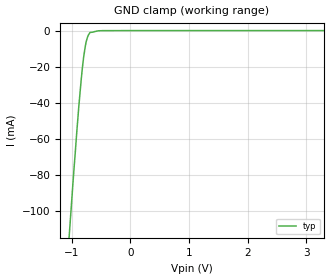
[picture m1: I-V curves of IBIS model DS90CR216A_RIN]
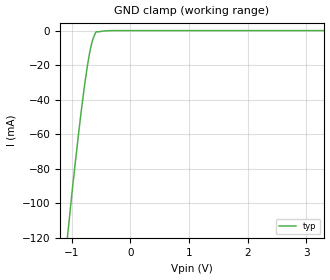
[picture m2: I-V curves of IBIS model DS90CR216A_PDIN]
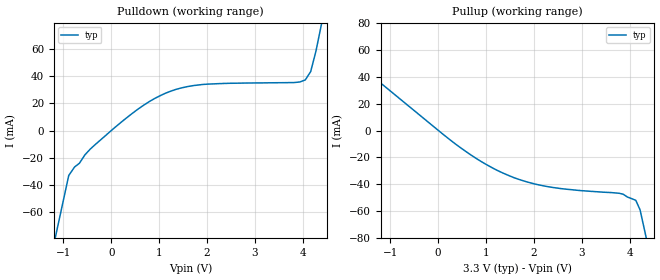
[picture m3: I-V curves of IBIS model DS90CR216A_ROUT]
|   National Semiconductor Corporation
|   Interface Products Group
|   IBIS Model of DS90CR216A
|   21-Bit LVDS Channel Link Receiver
|   48L TSSOP
[IBIS Ver]   2.1
[Comment char]  |_char
[File name]   90cr216a.ibs
[File Rev]   1.0
[Date]   10/07/04
[Source]   This is an empirical model.
[Notes]   File created by dglisic.
Rev. 1.0:
[Disclaimer]
(C) Copyright National Semiconductor Corporation 1994
   All rights reserved
   National Semiconductor Corporation hereby grants
the user of this IBIS model a non-exclusive, nontransferable
license to use this IBIS model under the following terms.
Before using this IBIS model, the user should read this
license.  If the user does not accept these terms,  the
IBIS model should be returned to National within 30 days.
   The user is granted this license only to use the
IBIS model and is not granted rights to sell, load, rent,
lease or license the IBIS model in whole or in part, or in
modified form to anyone other than user. User may modify
the IBIS model to suit its specific applications but rights
to derivative works and such modifications shall belong to
National.
   This IBIS model is provided on an "AS IS" basis and
National makes absolutely no warranty with respect to the
information contained herein.NATIONAL DISCLAIMS AND CUSTOMER
WAIVES ALL WARRANTIES, EXPRESS OR IMPLIED, INCLUDING
WARRANTIES OF MERCHANTABILITY OR FITNESS FOR A PARTICULAR
PURPOSE. The entire risk as to quality and performance is
with the Customer. ACCORDINGLY, IN NO EVENT SHALL THE
COMPANY BE LIABLE FOR ANY DAMAGES, WHETHER IN CONTRACT OR
TORT,INCLUDING ANY LOST PROFITS OR OTHER INCIDENTAL,
CONSEQUENTIAL, EXEMPLARY, OR PUNITIVE DAMAGES ARISING OUT
OF THE USE OR APPLICATION OF THE IBIS model provided in
this package.Further, National reserves the right to make
changes without notice to any product herein to improve
reliability, function, or design. National does not convey
any license under patent rights or any other intellectual
property rights, including those of third parties.
   National is not obligated to provide maintenance or support
for the licensed IBIS model.
Contact National at ATTN:INTERFACE APPLICATIONS/IBIS MODELS.
2900 Semiconductor Drive, M/S A2595, Santa Clara, CA 95052-8090
[Copyright]   Copyright 1994, National Semiconductor, All Rights Reserved
[Component]   DS90CR216AMTD
[Manufacturer]  National Semiconductor Corp
[Package]
|   typ   min   max
R_pkg   50.0m   50.0m   50.0m
L_pkg   1.49n   0.95n   2.07n
C_pkg   0.306p   0.146p   0.429p
[Pin]   signal_name   model_name   R_pin   L_pin   C_pin
1   RxOUT17   DS90CR216A_ROUT   50.0m   2.07n   0.429p
2   RxOUT18   DS90CR216A_ROUT   50.0m   1.49n   0.306p
3   GND   GND   50.0m   1.49n   0.146p
4   RxOUT19   DS90CR216A_ROUT   50.0m   0.95n   0.152p
5   RxOUT20   DS90CR216A_ROUT   50.0m   0.95n   0.152p
6   N/C   NC   50.0m   0.95n   0.146p
7   LVDSGND   GND   50.0m   1.49n   0.306p
8   RxIN0-   DS90CR216A_RIN   50.0m   2.07n   0.429p
9   RxIN0+   DS90CR216A_RIN   50.0m   2.07n   0.429p
10   RxIN1-   DS90CR216A_RIN   50.0m   1.49n   0.306p
11   RxIN1+   DS90CR216A_RIN   50.0m   0.95n   0.146p
12   LVDSVCC   POWER   50.0m   0.95n   0.152p
13   LVDSGND   GND   50.0m   0.95n   0.152p
14   RxIN2-   DS90CR216A_RIN   50.0m   0.95n   0.146p
15   RxIN2+   DS90CR216A_RIN   50.0m   1.49n   0.306p
16   RxCLKIN-   DS90CR216A_RIN   50.0m   2.07n   0.429p
17   RxCLKIN+   DS90CR216A_RIN   50.0m   2.07n   0.429p
18   LVDSGND   GND   50.0m   1.49n   0.306p
19   PLLGND   GND   50.0m   0.95n   0.146p
20   PLLVCC   POWER   50.0m   0.95n   0.152p
21   PLLGND   GND   50.0m   0.95n   0.152p
22   PWRDWN*   DS90CR216A_PDIN   50.0m   0.95n   0.146p
23   RxCLKOUT   DS90CR216A_ROUT   50.0m   1.49n   0.306p
24   RxOUT0   DS90CR216A_ROUT   50.0m   2.07n   0.429p
25   GND   GND   50.0m   2.07n   0.429p
26   RxOUT1   DS90CR216A_ROUT   50.0m   1.49n   0.306p
27   RxOUT2   DS90CR216A_ROUT   50.0m   0.95n   0.146p
28   VCC   POWER   50.0m   0.95n   0.152p
29   RxOUT3   DS90CR216A_ROUT   50.0m   0.95n   0.152p
30   RxOUT4   DS90CR216A_ROUT   50.0m   0.95n   0.146p
31   RxOUT5   DS90CR216A_ROUT   50.0m   1.49n   0.306p
32   GND   GND   50.0m   2.07n   0.429p
33   RxOUT6   DS90CR216A_ROUT   50.0m   2.07n   0.429p
34   RxOUT7   DS90CR216A_ROUT   50.0m   1.49n   0.306p
35   RxOUT8   DS90CR216A_ROUT   50.0m   0.95n   0.146p
36   VCC   POWER   50.0m   0.95n   0.152p
37   RxOUT9   DS90CR216A_ROUT   50.0m   0.95n   0.152p
38   GND   GND   50.0m   0.95n   0.146p
39   RxOUT10   DS90CR216A_ROUT   50.0m   1.49n   0.306p
40   RxOUT11   DS90CR216A_ROUT   50.0m   2.07n   0.429p
41   RxOUT12   DS90CR216A_ROUT   50.0m   2.07n   0.429p
42   VCC   POWER   50.0m   2.07n   0.429p
43   RxOUT13   DS90CR216A_ROUT   50.0m   1.49n   0.306p
44   GND   GND   50.0m   0.95n   0.146p
45   RxOUT14   DS90CR216A_ROUT   50.0m   0.95n   0.152p
46   RxOUT15   DS90CR216A_ROUT   50.0m   0.95n   0.152p
47   RxOUT16   DS90CR216A_ROUT   50.0m   0.95n   0.146p
48   VCC   POWER   50.0m   1.49n   0.306p
[Diff_pin]   inv_pin   vdiff   tdelay_typ   tdelay_min   tdelay_max
| The '+' pin is Diff_pin and the '-' pin is the inv_pin
9   8   .2   0 0 0
11   10   .2   0 0 0
15   14   .2   0 0 0
17   16   .2   0 0 0
| Models and submodels in the file (3): DS90CR216A_RIN (Input), DS90CR216A_PDIN (Input), DS90CR216A_ROUT (3-state)
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|   RECEIVER INPUT  MODEL
[Model]   DS90CR216A_RIN
Model_type   Input
|Signals   RxIN+,RxIN- ; RxCLKIN+, RxCLKIN-
Vinh = .1
Vinl = -.1
|   typ   min   max
C_comp   4.6931pF   4.6931pF   4.6931pF
|   typ   min   max
[Temperature Range]   25.0   85.0   -40.0
[Voltage range]   3.3V   3.0V   3.6V
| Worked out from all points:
|   GND clamp passes 1 mA (typ) near -0.67 V on its own axis
[Power_clamp]
| Note that the[POWER_clamp]voltage table is referenced to Vcc
| and is calculated using Vtable=Vcc - Vmeasured.
|Voltage   I(typ)   I(min)   I(max)
-3V       0A         NA         NA
0V        0A         NA         NA
[GND_clamp]
|Voltage   I(typ)   I(min)   I(max)
-3.3V     -1.145A    NA         NA
-1.001V   -93.37mA   NA         NA
-962.8mV  -76.1mA    NA         NA
-881.2mV  -41.82mA   NA         NA
-839.9mV  -26.91mA   NA         NA
-819.2mV  -20.28mA   NA         NA
-798.6mV  -14.57mA   NA         NA
-757.8mV  -6.396mA   NA         NA
-716mV    -2.36mA    NA         NA
-690.4mV  -1.091mA   NA         NA
-439.6mV  -28.58uA   NA         NA
3.3V      0A         NA         NA
|   RECEIVER PWRDWN* INPUT MODEL
[Model]   DS90CR216A_PDIN
Model_type   Input
|Signals   PWRDWN*
Vinh = 2.0
Vinl = 0.8
|   typ   min   max
C_comp   4.2707pF   4.2707pF   4.2707pF
|   typ   min   max
[Temperature Range]   25.0   85   -40
[Voltage range]   3.3V   3.0V   3.6V
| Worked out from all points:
|   GND clamp passes 1 mA (typ) near -0.59 V on its own axis
[GND_clamp]
|Voltage   I(typ)   I(min)   I(max)
-3.3V     -852.9mA   NA         NA
-1.002V   -95.17mA   NA         NA
-941.7mV  -76.32mA   NA         NA
-859.6mV  -52.18mA   NA         NA
-778.4mV  -30.47mA   NA         NA
-736.6mV  -20.8mA    NA         NA
-695.3mV  -12.71mA   NA         NA
-675.2mV  -9.298mA   NA         NA
-633.4mV  -4.243mA   NA         NA
-591mV    -870.7uA   NA         NA
-287.2mV  -7.856uA   NA         NA
3.3V      524nA      NA         NA
[Power_clamp]
| Note that the[POWER_clamp]voltage table is referenced to Vcc
| and is calculated using Vtable=Vcc - Vmeasured.
|Voltage   I(typ)   I(min)   I(max)
-3.3V     0A         0A         0A
0V        0A         0A         0A
|   RECEIVER OUTPUT  MODEL
[Model]   DS90CR216A_ROUT
Model_type   3-state
| Signals   RxOUT0 ~ RxOUT20
Vmeas = 1.5V   |This is 0.0v differential on output
Cref = 8pF   |Timing specification test load capacitance value
Vref = 0   |Timing specification test load voltage; GND
| variable   typ   min   max
C_comp   4.3866pF   4.3866pF   4.3866pF
|   typ   min   max
[Temperature Range]   25.0   85   -40
[Voltage range]   3.3V   3.0V   3.6V
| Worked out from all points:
|   slope of the pulldown table from 0 to 0.495 V, typ, clamps not added: 35.2 ohm
|   slope of the pullup table from 0 to 0.495 V, typ, clamps not added: 36.1 ohm
[Pulldown]
| Voltage   I(typ)   I(min)   I(max)
-3.3V     -424.5mA   NA         NA
-1.001V   -51.24mA   NA         NA
-888.6mV  -32.95mA   NA         NA
-439.6mV  -13.6mA    NA         NA
458.8mV   13.11mA    NA         NA
1.131V    27.37mA    NA         NA
1.917V    33.79mA    NA         NA
3.825V    35.19mA    NA         NA
4.049V    37.1mA     NA         NA
4.162V    43.2mA     NA         NA
4.383V    77.25mA    NA         NA
6.6V      501.2mA    NA         NA
[Pullup]
| Note that the[Pullup]voltage table is referenced to Vcc
| and is calculated using Vtable=Vcc - Vmeasured.
|Voltage   I(typ)   I(min)   I(max)
-3.3V     97.14mA    NA         NA
1.416mV   129.9uA    NA         NA
439.6mV   -12.14mA   NA         NA
790.7mV   -20.76mA   NA         NA
1.406V    -32.59mA   NA         NA
1.843V    -38.27mA   NA         NA
2.282V    -41.87mA   NA         NA
3.862V    -47.55mA   NA         NA
4.126V    -52.15mA   NA         NA
4.215V    -59.32mA   NA         NA
4.302V    -73.48mA   NA         NA
6.6V      -447.4mA   NA         NA
[GND_clamp]
| Outputs in Tri-state.
| Voltage   I(typ)   I(min)   I(max)
| Receiver output is non-tristable
-3V       0A         NA         NA
3V        0A         NA         NA
[POWER_clamp]
| Note that the[POWER_clamp]voltage table is referenced to Vcc
| and is calculated using Vtable=Vcc - Vmeasured.
| Outputs in Tri-state.
|Voltage   I(typ)   I(min)   I(max)
| Receiver output is non-tristable
-3V       0A         NA         NA
0V        0A         NA         NA
[Ramp]
| Note: Ramp rate measured on single-ended Driver Output.
|   typ   min   max
dV/dt_r   2.083/1.3643n   NA   NA
dV/dt_f   2.040/1.4065n   NA   NA
R_load = 1MOhm  | Represent Hi-Z
